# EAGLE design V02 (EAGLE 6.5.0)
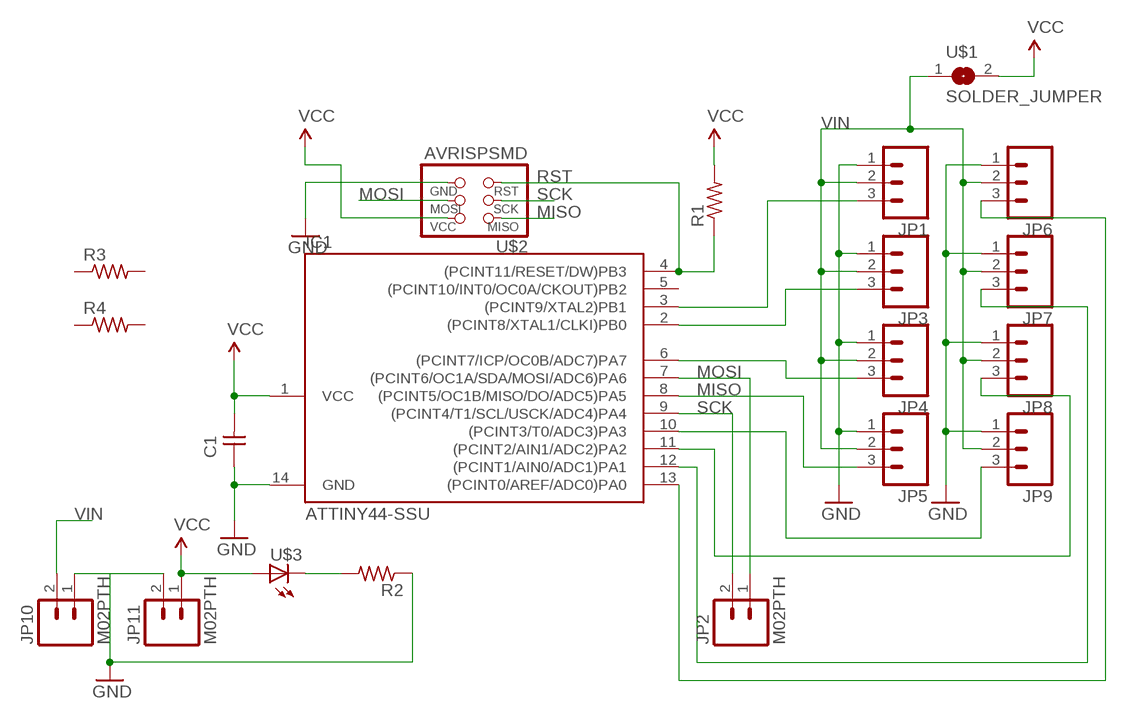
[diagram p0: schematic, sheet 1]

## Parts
C1  UNPOLARIZED_CAPACITOR1206  [1206]
IC1  ATTINY44-SSU  [SOIC14]
JP1  M03PTH  [1X03]
JP2  M02PTH  [1X02]
JP3  M03PTH  [1X03]
JP4  M03PTH  [1X03]
JP5  M03PTH  [1X03]
JP6  M03PTH  [1X03]
JP7  M03PTH  [1X03]
JP8  M03PTH  [1X03]
JP9  M03PTH  [1X03]
JP10  M02PTH  [1X02]
JP11  M02PTH  [1X02]
R1  RESISTOR1206  [1206]
R2  RESISTOR1206  [1206]
R3  RESISTOR1206  [1206]
R4  RESISTOR1206  [1206]
U$1  SOLDER_JUMPER  [SJFAB]
U$2  AVRISPSMD  [2X03SMD]
U$3  LED1206  [1206]

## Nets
GND: C1.1 IC1.14(GND) JP1.1 JP3.1 JP4.1 JP5.1 JP6.1 JP7.1 JP8.1 JP9.1 JP10.1 JP11.2 R2.1 U$2.6(GND)
MISO: IC1.8((PCINT5/OC1B/MISO/DO/ADC5)PA5) JP5.3 U$2.1(MISO)
MOSI: IC1.7((PCINT6/OC1A/SDA/MOSI/ADC6)PA6) JP2.1 U$2.4(MOSI)
N$1: IC1.6((PCINT7/ICP/OC0B/ADC7)PA7) JP4.3
N$2: IC1.10((PCINT3/T0/ADC3)PA3) JP9.3
N$3: IC1.11((PCINT2/AIN1/ADC2)PA2) JP8.3
N$4: IC1.12((PCINT1/AIN0/ADC1)PA1) JP7.3
N$5: IC1.13((PCINT0/AREF/ADC0)PA0) JP6.3
N$6: IC1.2((PCINT8/XTAL1/CLKI)PB0) JP3.3
N$7: IC1.3((PCINT9/XTAL2)PB1) JP1.3
N$8: R2.2 U$3.2(C)
RST: IC1.4((PCINT11/RESET/DW)PB3) R1.1 U$2.5(RST)
SCK: IC1.9((PCINT4/T1/SCL/USCK/ADC4)PA4) JP2.2 U$2.3(SCK)
VCC: C1.2 IC1.1(VCC) JP11.1 R1.2 U$1.2 U$2.2(VCC) U$3.1(A)
VIN: JP1.2 JP3.2 JP4.2 JP5.2 JP6.2 JP7.2 JP8.2 JP9.2 JP10.2 U$1.1
Unconnected: IC1.5((PCINT10/INT0/OC0A/CKOUT)PB2) R3.1 R3.2 R4.1 R4.2

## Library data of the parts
C1 = ng:UNPOLARIZED_CAPACITOR: unpolarized_capacitor
IC1 = fab:ATTINY44
JP1 JP3-JP9 = SparkFun-Connectors:M03: Header 3 Standard 3-pin 0.1" header. Use with straight break away headers (SKU : PRT-00116), right angle break away headers (PRT-00553), swiss pins (PRT-00743), machine pins (PRT-00117), and female headers (PRT-00115). Molex polarized connector foot print use with SKU : PRT-08232 with associated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
JP2 JP10 JP11 = SparkFun-Connectors:M02: Standard 2-pin 0.1" header. Use with
R1-R4 = ng:RESISTOR
U$1 = fab:SOLDER_JUMPER
U$2 = fab:AVRISP
U$3 = ng:LED

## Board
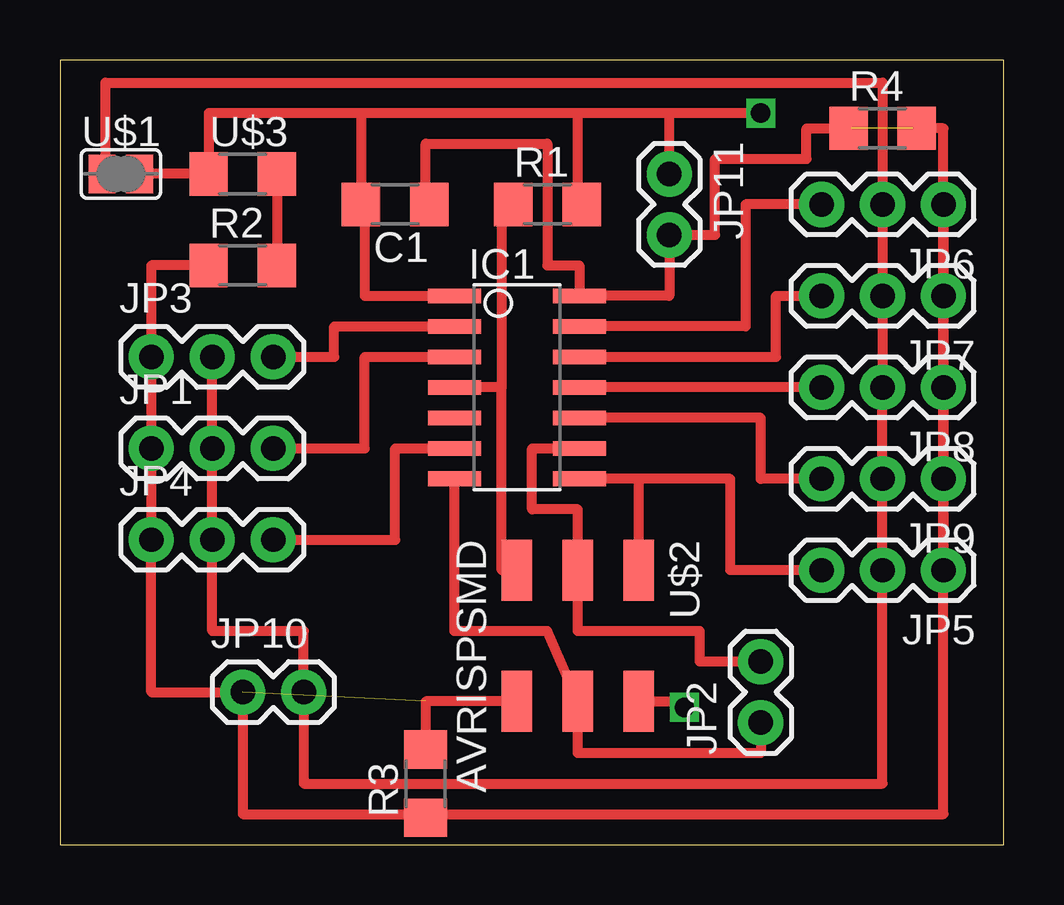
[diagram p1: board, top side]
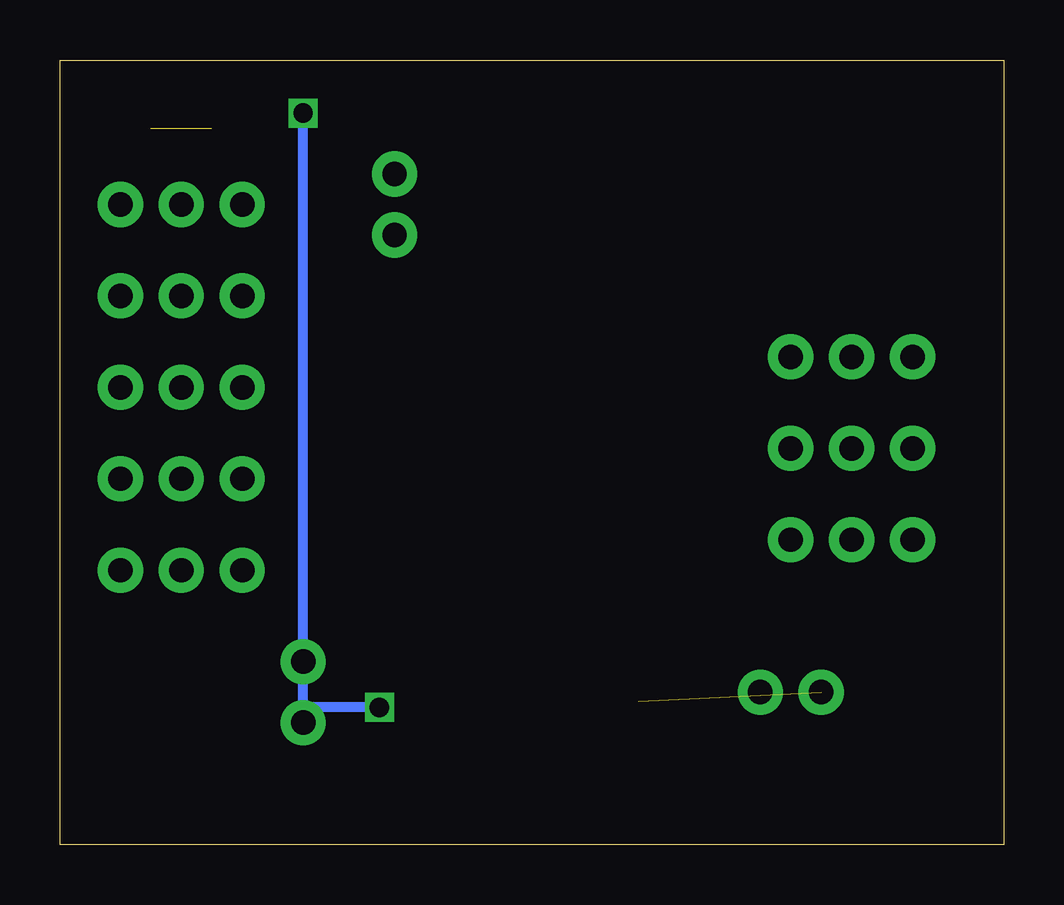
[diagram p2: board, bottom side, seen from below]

Size 39.35 x 32.69 mm. Coordinates in mm from the lower left corner, seen from the top.
Outline: 0,0 39.35,0 39.35,32.69 0,32.69 0,0
Copper layers (1*16): Top 0.035mm / dielectric 1.5mm / Bottom 0.035mm
Design rules "default *": minimum track width 10mil, minimum drill 24mil, track to track 17mil, track to pad 17mil, pad to pad 8mil, via to via 8mil, smd to smd 8mil, copper to edge 40mil, drill to drill 8mil, minimum pad ring 10mil, minimum via ring 8mil, stop-mask expansion 4mil, vias tented up to drill 0mil, thermal gap 10mil

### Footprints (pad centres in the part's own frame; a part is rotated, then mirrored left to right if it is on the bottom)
1206 = smd 1.6 x 1.803: 1 -1.422,0; 2 1.422,0
SOIC14 = smd 0.61 x 2.21: 1 -3.81,-2.603; 2 -2.54,-2.603; 3 -1.27,-2.603; 4 0,-2.603; 5 1.27,-2.603; 6 2.54,-2.603; 7 3.81,-2.603; 8 3.81,2.603; 9 2.54,2.603; 10 1.27,2.603; 11 0,2.603; 12 -1.27,2.603; 13 -2.54,2.603; 14 -3.81,2.603
1X03 = drill 1.016 pad 1.88: 1 0,0; 2 2.54,0; 3 5.08,0
1X02 = drill 1.016 pad 1.88: 1 0,0; 2 2.54,0
SJFAB = smd 1.118 x 1.6: 1 -0.787,0; 2 0.787,0
2X03SMD = smd 2.54 x 1.27: 1 -2.54,2.54; 2 2.92,2.54; 3 -2.54,0; 4 2.92,0; 5 -2.54,-2.54; 6 2.92,-2.54

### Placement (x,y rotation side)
C1  13.97,26.67 180 top
IC1  19.05,19.05 270 top
JP1  3.81,16.51 0 top
JP2  29.21,5.08 90 top
JP3  3.81,20.32 0 top
JP4  3.81,12.7 0 top
JP5  36.83,11.43 180 top
JP6  36.83,26.67 180 top
JP7  36.83,22.86 180 top
JP8  36.83,19.05 180 top
JP9  36.83,15.24 180 top
JP10  7.62,6.35 0 top
JP11  25.4,27.94 270 top
R1  20.32,26.67 0 top
R2  7.62,24.13 0 top
R3  15.24,2.54 90 top
R4  34.29,29.84 0 top
U$1  2.54,27.94 0 top
U$2  21.59,8.89 270 top
U$3  7.62,27.94 0 top

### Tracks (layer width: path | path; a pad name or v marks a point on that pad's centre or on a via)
GND  (2 unrouted)
  Top 0.406: JP3.1 JP1.1 JP4.1 | JP5.1 JP9.1 JP8.1 JP7.1 JP6.1 JP5.1 | C1.1 15.24,26.67 15.24,29.21 20.32,29.21 20.32,24.13 21.65,24.13 IC1.14 25.4,22.86 JP11.2 27.3,25.4 27.3,28.57 31.11,28.57 31.11,29.84 33.02,29.84 | JP5.1 36.83,1.27 7.62,1.27 JP10.1 3.81,6.35 JP4.1 | JP3.1 3.81,24.13 R2.1 | JP3.1 JP4.1 | U$2.6 15.24,5.97 15.24,3.81 | JP5.1 36.83,29.84 35.56,29.84
MISO
  Top 0.406: JP5.3 27.94,11.43 27.94,15.24 24.13,15.24 | 24.13,15.24 IC1.8 | U$2.1 24.13,15.24
MOSI
  Top 0.406: IC1.7 16.45,8.89 20.32,8.89 U$2.4 21.59,3.81 29.21,3.81 JP2.1
N$1
  Top 0.406: JP4.3 13.97,12.7 13.97,16.51 IC1.6
N$2
  Top 0.406: JP9.3 29.21,15.24 29.21,17.78 IC1.10
N$3
  Top 0.406: JP8.3 IC1.11
N$4
  Top 0.406: IC1.12 29.84,20.32 29.84,22.86 JP7.3
N$5
  Top 0.406: JP6.3 28.57,26.67 28.57,21.59 IC1.13
N$6
  Top 0.406: JP3.3 11.43,20.32 11.43,21.59 IC1.2
N$7
  Top 0.406: JP1.3 12.7,16.51 12.7,20.32 IC1.3
N$8
  Top 0.406: U$3.2 R2.2
RST
  Top 0.406: U$2.5 18.41,11.43 18.41,19.05 | 18.41,19.05 IC1.4 | R1.1 18.41,26.67 18.41,19.05
SCK
  Top 0.406: IC1.9 19.68,16.51 19.68,13.97 21.59,13.97 U$2.3 21.59,8.89 26.67,8.89 26.67,7.62 JP2.2
VCC  (via drill 0.8)
  Top 0.406: R1.2 21.59,26.67 21.59,30.48 | 21.59,30.48 12.55,30.48 | 12.55,30.48 C1.2 12.7,26.67 12.7,22.86 IC1.1 | U$1.2 U$3.1 6.2,30.48 12.55,30.48 | JP11.1 25.4,30.48 | 25.4,30.48 21.59,30.48 | U$2.2 26.04,5.97 v26.04,5.71 | v29.21,30.48 25.4,30.48
  Bottom 0.406: v26.04,5.71 29.21,5.71 v29.21,30.48
VIN
  Top 0.406: JP3.2 JP1.2 JP4.2 6.35,8.89 10.16,8.89 JP10.2 10.16,2.54 34.29,2.54 JP5.2 JP9.2 JP8.2 JP7.2 JP6.2 34.29,31.75 1.91,31.75 1.91,27.94 U$1.1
